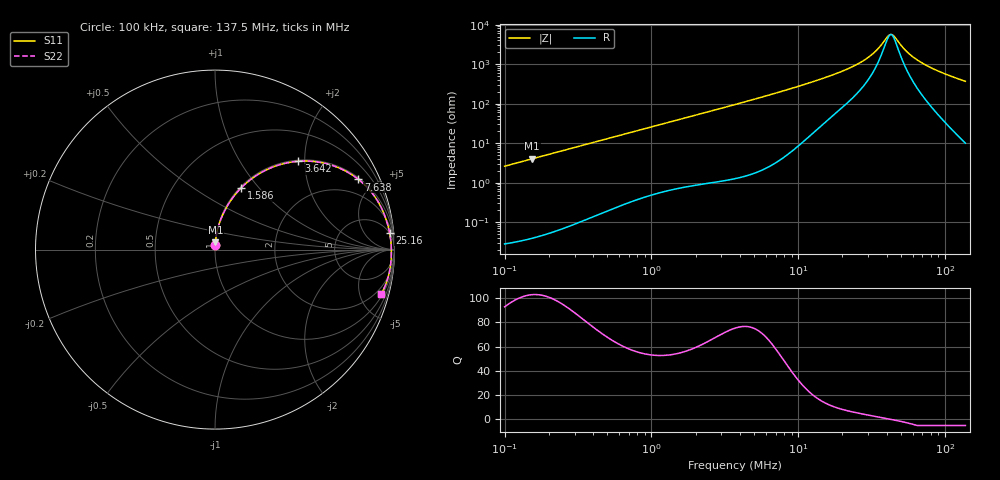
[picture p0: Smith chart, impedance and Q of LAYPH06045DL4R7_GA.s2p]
! LAYPH06045DL4R7_GA  S-PARAMETER MODEL  ( General Type )
! Model Generated by TAIYO YUDEN Corporation (http://www.ty-top.com)
! Version 2.0
! TAIYO YUDEN Control No. 180914NI43SB-FBB
! Copyright(c) 2018 TAIYO YUDEN CO.,LTD. All Rights Reserved.
! Product Description (link to TY-COMPAS)
! https://ds.yuden.co.jp/TYCOMPAS/or/detail?pn=LAYPH06045DL4R7NGA&u=M
! Products Name : Inductors
! Characteristics :
!  Inductance : 4.7 uH , SRF(min) : -Hz , DC Resistance(max) : 0.026 Ohm
!  Rated Current : Saturation :3.1 A , Temp Rise : 2.3 A (25 degC)
!  Case Size : 6.3 x 6.0 / 0.248 x 0.236 [mm/inch] , Thickness : 4.5 / 0.177 [mm/inch]
!  (Conditions: Temperature = 25 degC , DC Bias Current/Voltage = 0A / 0V)
! External Node Assignments :
!  1  o---GGG---o  2
! GND o---------o GND
! Frequency Range : 0.1MHz  -  137.487582MHz  [ 402 STEP ]
# MHz S RI R 50
! Freq[MHz].  S11 Real  S11 Imag  S21 Real  S21 Imag  S12 Real  S12 Imag  S22 Real  S22 Imag
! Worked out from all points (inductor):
!   401 points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, 100 kHz to 137.5 MHz, reference 50 ohm
!   read as one part in series: L = 4.15 uH near 103.7 kHz
!   highest Q = 103 at 154.3 kHz (marker M1), where L = 4.15 uH
!   self-resonance near 42.49 MHz
!   S11 on the Smith chart (normalised r, x): 100 kHz: 1.00, +0.05; 1.586 MHz: 1.01, +0.81; 3.642 MHz: 1.02, +1.86; 7.638 MHz: 1.08, +4.05; 25.16 MHz: 5, +19; 137.5 MHz: 1.20, -7.35
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0.1  0.000961 0.0261  0.999 -0.0261  0.999 -0.0261  0.000961 0.0261
0.154275  0.00201 0.0401  0.998 -0.0401  0.998 -0.0401  0.00201 0.0401
0.335474  0.00859 0.0865  0.9914 -0.0865  0.9914 -0.0865  0.00859 0.0865
0.631331  0.0285 0.1584  0.9715 -0.1584  0.9715 -0.1584  0.0285 0.1584
1.125429  0.0813 0.264  0.9187 -0.264  0.9187 -0.264  0.0813 0.264
1.586302  0.1457 0.3438  0.8543 -0.3438  0.8543 -0.3438  0.1457 0.3438
2.360425  0.269 0.4357  0.731 -0.4357  0.731 -0.4357  0.269 0.4357
3.641548  0.465 0.4921  0.535 -0.4921  0.535 -0.4921  0.465 0.4921
3.707932  0.474 0.4927  0.526 -0.4927  0.526 -0.4927  0.474 0.4927
5.226359  0.6442 0.472  0.3558 -0.472  0.3558 -0.472  0.6442 0.472
7.637621  0.7994 0.391  0.2006 -0.391  0.2006 -0.391  0.7994 0.391
12.43915  0.9157 0.2546  0.0843 -0.2546  0.0843 -0.2546  0.9157 0.2546
18.84695  0.9579 0.1532  0.0421 -0.1532  0.0421 -0.1532  0.9579 0.1532
25.16353  0.9726 0.0948  0.0274 -0.0948  0.0274 -0.0948  0.9726 0.0948
32.40491  0.9797 0.0483  0.0203 -0.0483  0.0203 -0.0483  0.9797 0.0483
41.73016  0.9825 0.00415  0.0175 -0.00415  0.0175 -0.00415  0.9825 0.00415
43.26546  0.9827 -0.0021  0.0173 0.0021  0.0173 0.0021  0.9827 -0.0021
44.85725  0.9827 -0.00836  0.0173 0.00836  0.0173 0.00836  0.9827 -0.00836
55.71608  0.9818 -0.0466  0.0182 0.0466  0.0182 0.0466  0.9818 -0.0466
69.20356  0.978 -0.0875  0.022 0.0875  0.022 0.0875  0.978 -0.0875
94.08159  0.9647 -0.1533  0.0353 0.1533  0.0353 0.1533  0.9647 -0.1533
137.4876  0.9252 -0.2497  0.0748 0.2497  0.0748 0.2497  0.9252 -0.2497
